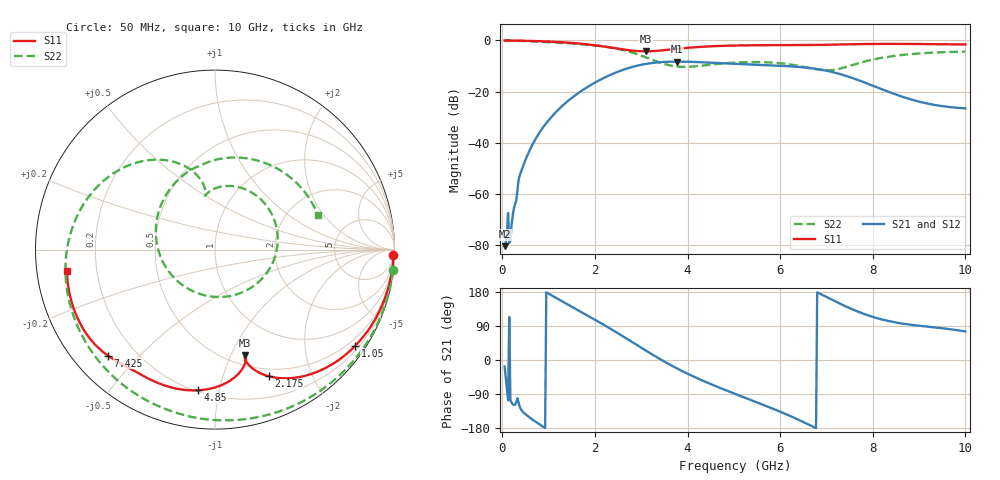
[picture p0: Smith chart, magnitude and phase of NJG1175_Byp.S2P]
! Created Fri Jun 18 20:05:49 2021
# hz S ma R 50
! 2 Port Network Data from SP1.SP block
! freq  magS11  angS11  magS21  angS21  magS12  angS12  magS22  angS22
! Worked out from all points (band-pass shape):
!   399 points, 50 MHz to 10 GHz, reference 50 ohm
!   highest |S21| = -8.27 dB at 3.775 GHz (marker M1); lowest = -80.4 dB at 50 MHz (marker M2)
!   |S21| within 3 dB of the highest: 2.641 GHz to 6.835 GHz (4.194 GHz wide, 88.5 % of centre)
!   lowest |S11| = -4.2 dB at 3.1 GHz (marker M3), VSWR 4.17, Z = 30 - j56.6 ohm
!   |S11| at or under -10 dB: nowhere
!   |S22| runs from -11.7 to 0.0 dB; largest |S21 - S12| = 0.00054
!   S11 on the Smith chart (normalised r, x): 50 MHz: 13, -66; 1.05 GHz: 0.31, -3.20; 2.175 GHz: 0.42, -1.43; 4.85 GHz: 0.21, -0.87; 7.425 GHz: 0.10, -0.41; 10 GHz: 0.09, -0.07
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5e7  0.9944 -1.7  9.581e-05 -17.3  9.582e-05 -17.3  0.9997 -6.6
1e8  0.994 -3.3  0.0001743 -73.9  0.0001744 -73.9  0.9985 -13.1
1.25e8  0.9938 -4.1  0.0004266 -106.4  0.0004267 -106.4  0.9969 -16.5
1.5e8  0.9935 -5.0  0.0001109 113.5  0.000111 113.5  0.9962 -19.4
1.75e8  0.9932 -5.8  0.0001239 -106.7  0.0001239 -106.7  0.9959 -22.7
2.25e8  0.9923 -7.4  0.0003752 -117.3  0.0003753 -117.3  0.9938 -29.1
4e8  0.9877 -13.2  0.002662 -129.6  0.002662 -129.6  0.9828 -50.9
7e8  0.974 -23.0  0.01111 -161.3  0.01111 -161.3  0.9549 -84.9
1.05e9  0.9476 -34.4  0.0311 171.7  0.0311 171.7  0.9177 -118.7
1.725e9  0.8588 -55.3  0.1057 125.4  0.1057 125.4  0.8424 -171.4
2.175e9  0.7658 -67.1  0.182 94.1  0.182 94.1  0.7659 158.2
2.625e9  0.6634 -73.9  0.2701 61.0  0.27 61.0  0.6427 130.3
3.1e9  0.6131 -74.2  0.348 24.8  0.348 24.8  0.4686 107.2
3.375e9  0.6306 -74.1  0.3739 4.6  0.3738 4.6  0.3781 100.5
3.775e9  0.6862 -77.5  0.3859 -22.5  0.3859 -22.4  0.309 99.8
4.85e9  0.7893 -96.8  0.3555 -80.9  0.3554 -80.8  0.3605 79.7
5.025e9  0.7961 -100.0  0.3494 -89.3  0.3493 -89.2  0.3694 72.2
6.025e9  0.8087 -116.6  0.3188 -137.6  0.3187 -137.5  0.3574 12.4
6.7e9  0.8142 -125.7  0.2847 -175.4  0.2847 -175.3  0.2819 -57.9
7.425e9  0.8393 -135.2  0.2028 140.9  0.2028 141.0  0.3037 -170.9
8.35e9  0.8569 -148.9  0.09856 102.7  0.09857 102.8  0.4803 97.9
1e10  0.834 -171.7  0.04714 75.3  0.04709 75.3  0.6045 18.4
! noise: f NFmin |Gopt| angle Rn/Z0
5e+07  31.06  0.9898  1.604  7.9e+04
1.15e+09  27.48  0.4884  177.3  92.99
2.25e+09  26.45  0.8956  -169.3  34.8
3.35e+09  28.72  0.9386  -162.2  165.7
4.45e+09  31.83  0.9332  -154.3  598.2
5.575e+09  33.97  0.9298  -144.7  1719
6.675e+09  35.35  0.898  -130.5  4356
7.775e+09  41.48  0.5239  -101.1  1.157e+04
8.875e+09  50.15  0.2818  126.3  3.237e+04
1e+10  57.2  0.6015  159.9  5.68e+04
